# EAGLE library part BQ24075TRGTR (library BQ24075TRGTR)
1.5A USB-Friendly Li-Ion Battery Charger and Power-Path Management IC with 4.2 VBAT Source: Datasheet
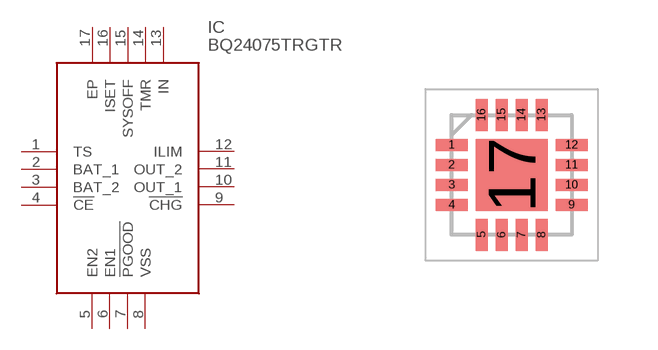
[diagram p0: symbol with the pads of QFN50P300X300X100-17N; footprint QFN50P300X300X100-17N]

Designator prefix IC

## BQ24075TRGTR (Description: 1.5A USB-Friendly Li-Ion Battery Charger and Power-Path Management IC with 4.2 VBAT; Height: 1mm; Manufacturer_Name: Texas Instruments; Manufacturer_Part_Number: BQ24075TRGTR; Mouser_Part_Number: 595-BQ24075TRGTR; Mouser_Price-Stock: https://www.mouser.co.uk/ProductDetail/Texas-Instruments/BQ24075TRGTR?qs=%2Fqzd9s%252BcLd4uxZAT5jNskQ%3D%3D)  [QFN50P300X300X100-17N]
1  TS
2  BAT_1
3  BAT_2
4  !CE
5  EN2
6  EN1
7  !PGOOD
8  VSS
9  !CHG
10  OUT_1
11  OUT_2
12  ILIM
13  IN
14  TMR
15  SYSOFF
16  ISET
17  EP

## Footprint QFN50P300X300X100-17N (pad centres in mm)
RGT(PVQFN-16)
smd 0.8 x 0.3: 1 -1.5,0.75; 2 -1.5,0.25; 3 -1.5,-0.25; 4 -1.5,-0.75; 9 1.5,-0.75; 10 1.5,-0.25; 11 1.5,0.25; 12 1.5,0.75
smd 0.3 x 0.8: 5 -0.75,-1.5; 6 -0.25,-1.5; 7 0.25,-1.5; 8 0.75,-1.5; 13 0.75,1.5; 14 0.25,1.5; 15 -0.25,1.5; 16 -0.75,1.5
smd 1.8 x 1.8: 17 0,0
